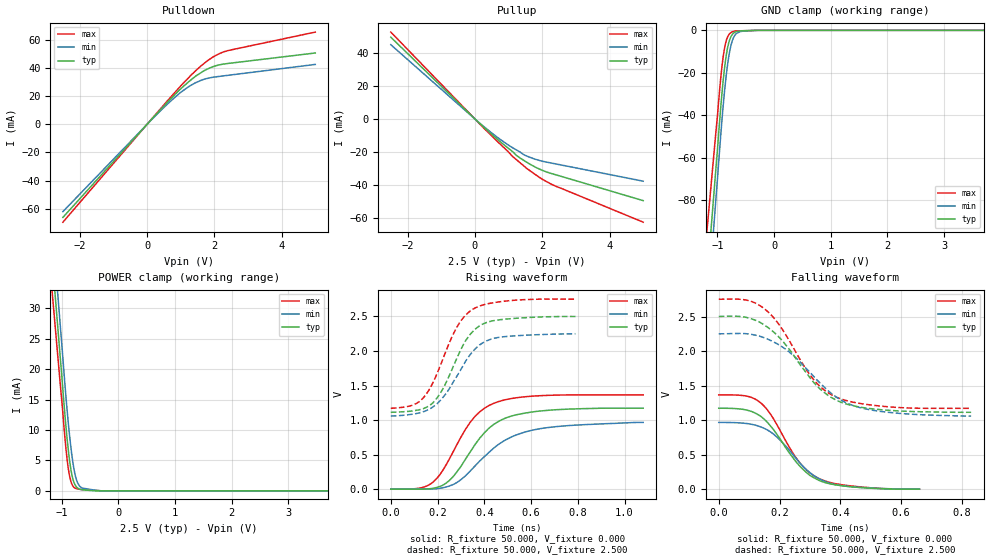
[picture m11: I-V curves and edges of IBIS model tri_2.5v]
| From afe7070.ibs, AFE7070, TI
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[Model]   tri_2.5v
Model_type 3-state
Vref=0.000E+00
Rref=1.000E+06
Cref=0.000E+00
Vmeas=1.250E+00
C_comp   4.840E-13   4.750E-13   4.930E-13
[Voltage Range]   2.500E+00   2.250E+00   2.750E+00
[POWER Clamp Reference]   2.500E+00   2.250E+00   2.750E+00
[GND Clamp Reference]   0.000E+00   0.000E+00   0.000E+00
[Pullup Reference]   2.500E+00   2.250E+00   2.750E+00
[Pulldown Reference]   0.000E+00   0.000E+00   0.000E+00
[Temperature Range]   25   85   -40
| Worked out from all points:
|   slope of the pulldown table from 0 to 0.375 V, typ, clamps not added: 38.2 ohm
|   slope of the pullup table from 0 to 0.375 V, typ, clamps not added: 53.3 ohm
|   GND clamp passes 1 mA (typ) near -0.70 V on its own axis
|   POWER clamp passes 1 mA (typ) near -0.76 V on its own axis
|   rising waveform, R_fixture 50.000, V_fixture 0.000: 20-80 % time 161ps typ, 208ps min, 149ps max; typ from 0 V to 1.17 V
|   falling waveform, R_fixture 50.000, V_fixture 0.000: 20-80 % time 124ps typ, 128ps min, 120ps max; typ from 1.17 V to 0 V
|   rising waveform, R_fixture 50.000, V_fixture 2.500: 20-80 % time 124ps typ, 141ps min, 128ps max; typ from 1.11 V to 2.5 V
|   falling waveform, R_fixture 50.000, V_fixture 2.500: 20-80 % time 156ps typ, 175ps min, 144ps max; typ from 2.5 V to 1.11 V
[GND Clamp]
-2.5V     -559.2mA   -596.9mA   -482.2mA
-1.02V    -62.78mA   -77.07mA   -45.88mA
-940mV    -35.74mA   -48.82mA   -21.98mA
-900mV    -24mA      -35.96mA   -12.7mA
-880mV    -19.02mA   -30.17mA   -9.212mA
-820mV    -8.124mA   -15.92mA   -3.068mA
-780mV    -4.138mA   -9.346mA   -1.452mA
-740mV    -2.002mA   -5.086mA   -721uA
-680mV    -702.1uA   -1.881mA   -302.2uA
-600mV    -315.1uA   -628.6uA   -231.3uA
-280mV    0A         0A         0A
5V        0A         0A         0A
[Power Clamp]
-2.5V     189.6mA    199.8mA    174mA
-2.46V    185.1mA    194.8mA    169.4mA
-1.02V    21.48mA    26.74mA    17.15mA
-940mV    12.32mA    17.33mA    8.54mA
-900mV    8.299mA    12.97mA    4.932mA
-880mV    6.546mA    10.97mA    3.553mA
-820mV    2.682mA    5.936mA    1.139mA
-760mV    955.2uA    2.587mA    449uA
-720mV    477.6uA    1.366mA    324.7uA
-640mV    191.6uA    479.4uA    215.5uA
-280mV    0A         0A         0A
5V        0A         0A         0A
[Pullup]
-2.5V     49.56mA    45.02mA    52.66mA
260mV     -4.9mA     -4.526mA   -5.459mA
840mV     -15.25mA   -13.62mA   -16.91mA
1.1V      -19.42mA   -17.16mA   -22.29mA
1.24V     -22.15mA   -18.82mA   -24.74mA
1.44V     -24.92mA   -21.47mA   -28.19mA
1.86V     -29.8mA    -24.77mA   -34.57mA
2.28V     -33.05mA   -26.71mA   -39.58mA
5V        -49.44mA   -37.66mA   -62.5mA
[Pulldown]
-2.5V     -66.25mA   -62.13mA   -69.66mA
140mV     3.741mA    3.488mA    3.947mA
600mV     15.6mA     14.35mA    16.63mA
1V        25.3mA     22.79mA    27.35mA
1.26V     30.77mA    27.2mA     33.84mA
1.46V     34.63mA    29.86mA    38.55mA
1.68V     37.97mA    32.03mA    43.1mA
1.94V     40.92mA    33.5mA     47.67mA
2.28V     42.99mA    34.57mA    51.66mA
5V        50.86mA    42.71mA    65.74mA
[Rising Waveform]
R_fixture = 50.000
V_fixture = 0.000
V_fixture_min = 0.000
V_fixture_max = 0.000
|  time   V(typ)   V(min)   V(max)
0s        0V         0V         0V
150ps     1.609mV    -257uV     40.11mV
190ps     18.35mV    4.763mV    131.5mV
230ps     71.69mV    24.97mV    313.1mV
280ps     236.8mV    90.26mV    626.7mV
340ps     539.4mV    263.4mV    969mV
440ps     936.5mV    592.6mV    1.242V
520ps     1.062V     762.1mV    1.314V
640ps     1.131V     875.9mV    1.353V
1.08ns    1.172V     966.6mV    1.364V
[Falling Waveform]
R_fixture = 50.000
V_fixture = 0.000
V_fixture_min = 0.000
V_fixture_max = 0.000
|  time   V(typ)   V(min)   V(max)
0s        1.172V     966.6mV    1.364V
90ps      1.147V     951.6mV    1.349V
140ps     1.049V     898.7mV    1.243V
160ps     967.6mV    856.8mV    1.148V
190ps     801.5mV    759.8mV    944.3mV
260ps     366.7mV    414.9mV    419.3mV
290ps     234.9mV    275.5mV    271.9mV
330ps     127mV      151.7mV    153.5mV
420ps     41.86mV    41.83mV    54.66mV
660ps     0V         0V         0V
[Rising Waveform]
R_fixture = 50.000
V_fixture = 2.500
V_fixture_min = 2.250
V_fixture_max = 2.750
|  time   V(typ)   V(min)   V(max)
0s        1.113V     1.058V     1.171V
110ps     1.142V     1.095V     1.241V
150ps     1.181V     1.135V     1.367V
180ps     1.249V     1.19V      1.54V
220ps     1.436V     1.317V     1.86V
280ps     1.875V     1.621V     2.329V
350ps     2.279V     1.99V      2.603V
400ps     2.4V       2.13V      2.672V
460ps     2.45V      2.196V     2.71V
790ps     2.5V       2.25V      2.75V
[Falling Waveform]
R_fixture = 50.000
V_fixture = 2.500
V_fixture_min = 2.250
V_fixture_max = 2.750
|  time   V(typ)   V(min)   V(max)
0s        2.5V       2.25V      2.75V
90ps      2.488V     2.251V     2.739V
150ps     2.376V     2.192V     2.612V
200ps     2.194V     2.085V     2.373V
310ps     1.556V     1.643V     1.597V
350ps     1.389V     1.464V     1.426V
390ps     1.282V     1.323V     1.327V
450ps     1.2V       1.2V       1.253V
530ps     1.152V     1.127V     1.204V
830ps     1.113V     1.058V     1.171V
[Ramp]
dV/dt_r   6.9200E-01/1.6090E-10   5.6700E-01/2.0820E-10   8.0400E-01/1.4870E-10
dV/dt_f   8.3100E-01/1.5640E-10   7.1500E-01/1.7540E-10   9.4865E-01/1.4369E-10
R_load = 50
